| IBIS file generated by GenIBIS.pl Version 3.07
|   am35xxzer
[IBIS ver]   4.1
[File name]   sprm504.ibs
[File Rev]   1.0
[Date]   Mon May 10, 2010, 10:47:13
[Source]   Data created at Texas Instruments
[Notes]   1) IBIS spec conformance checker (IBISCK4) ran with 0 errors
   and 179 warnings.  Warnings can be waived.
[Disclaimer] Please be aware that in the absence of a written agreement,
   Texas Instruments (TI) assumes no liability for: 1) the
   accuracy of the IBIS models provided to your company, 2) the
   proper functioning of these IBIS models in your design or for
   any resulting applications, or, 3) infringement of patents,
   copyrights, or intellectual property rights resulting from
   your use of these IBIS models. TI provides IBIS models as a
   service to our customers and therefore reserves the right to
   limit distribution of the IBIS models.
[Copyright]   Property of Texas Instruments Incorporated. Unauthorised
   reproduction and/or distribution is strictly prohibited. This
   product is protected under copyright law and trade secret law
   as an unpublished work. Created 2010,(C) Copyright 2010,
   Texas Instruments Incorporated., All Rights Reserved. These
   commodities are under the U.S. Government distribution license
   control.As such,they are not to be re-exported without the
   prior approval of the U.S. Department of Commerce.
|   Component am35xxzer
[Component]   am35xxzer
[Manufacturer]   Texas Instruments.
[Package]
|   typ   min   max
R_pkg   0.33395   214.1400E-3   453.7600E-3
L_pkg   6.28345E-009   3.3793E-9   9.1876E-9
C_pkg   2.39255E-012   1.3394E-12   3.4457E-12
[Pin]   signal_name   model_name   R_pin   L_pin   C_pin
A2   MCBSP4_DX   Selector_25  394.1900E-3 7.9895E-9  1.9401E-12
A3   MCBSP4_CLKX   Selector_25  371.6000E-3 7.7376E-9  1.9311E-12
A4   MCBSP3_FSX   Selector_25  347.7300E-3 7.0891E-9  2.0982E-12
A5   UART2_CTS   Selector_12  328.5900E-3 6.4462E-9  1.5188E-12
A7   USB0_DRVVBUS   Selector_9   336.2200E-3 6.8852E-9  1.6105E-12
A8   SYS_32K   Selector_17  296.9800E-3 5.8091E-9  1.6649E-12
A10   SYS_XTALIN   Selector_11  282.6900E-3 5.0981E-9  1.6542E-12
A12   JTAG_TMS_TMSC   Selector_14  324.6800E-3 6.3416E-9  1.5318E-12
A13   DSS_DATA20   Selector_8   341.4400E-3 6.7413E-9  1.6482E-12
A14   DSS_DATA17   Selector_8   333.0200E-3 6.8421E-9  1.5875E-12
A15   DSS_DATA16   Selector_8   314.2700E-3 6.1729E-9  1.5039E-12
A16   DSS_DATA13   Selector_8   297.6500E-3 5.9252E-9  1.5015E-12
A17   DSS_DATA4   Selector_25  346.9100E-3 7.2431E-9  1.7900E-12
A18   DSS_DATA2   Selector_25  329.7600E-3 6.8073E-9  1.6863E-12
A19   DSS_DATA1   Selector_25  330.6900E-3 6.8826E-9  1.7355E-12
A20   DSS_DATA0   Selector_25  315.8500E-3 6.5578E-9  1.8340E-12
AA2   SDRC_D28   Selector_16  343.2000E-3 6.9062E-9  1.8222E-12
AA3   SDRC_D29   Selector_16  324.2800E-3 6.4573E-9  1.8291E-12
AA4   SDRC_D30   Selector_16  316.2700E-3 6.3226E-9  1.7135E-12
AA5   GPMC_A4   Selector_2   329.6700E-3 6.0019E-9  1.5140E-12
AA6   GPMC_A7   Selector_27  298.1300E-3 6.0001E-9  1.5038E-12
AA7   GPMC_D0   Selector_27  320.6800E-3 6.0389E-9  1.5462E-12
AA8   GPMC_D5   Selector_27  323.1800E-3 5.8436E-9  1.5422E-12
AA9   GPMC_D3   Selector_27  380.0900E-3 7.6125E-9  1.7128E-12
AA10   GPMC_D12   Selector_27  301.4100E-3 5.4391E-9  1.4352E-12
AA11   GPMC_NCS4   Selector_27  374.8300E-3 7.1356E-9  1.5639E-12
AA12   GPMC_NCS6   Selector_27  374.6200E-3 7.0731E-9  1.6544E-12
AA13   UART3_RX_IRRX   Selector_18  314.2500E-3 5.8029E-9  1.6148E-12
AA14   GPMC_NADV_ALE   Selector_20  353.2500E-3 6.2559E-9  1.6326E-12
AA15   GPMC_NWE   Selector_21  385.0100E-3 7.2004E-9  1.5876E-12
AA16   GPMC_WAIT1   Selector_22  399.6800E-3 7.9386E-9  1.7244E-12
AA17   I2C1_SCL   Selector_7   370.5100E-3 7.2651E-9  1.7713E-12
AA18   SYS_NRESPWRON   Selector_23  360.3900E-3 7.0919E-9  1.8556E-12
AA19   SYS_BOOT3   Selector_26  384.4600E-3 7.6592E-9  1.9352E-12
AA20   SYS_BOOT7   Selector_24  393.7300E-3 7.7930E-9  1.9516E-12
AA21   CCDC_FIELD   Selector_25  398.4600E-3 8.0595E-9  2.0452E-12
AB2   SDRC_D31   Selector_16  334.8800E-3 7.1146E-9  1.7302E-12
AB3   SDRC_DM3   Selector_28  329.7900E-3 6.8551E-9  1.7153E-12
AB4   GPMC_A3   Selector_2   347.2000E-3 6.7527E-9  1.4825E-12
AB5   GPMC_A5   Selector_2   343.8700E-3 6.4609E-9  1.5166E-12
AB6   GPMC_A6   Selector_27  346.1000E-3 6.4915E-9  1.5619E-12
AB7   GPMC_A9   Selector_27  311.5600E-3 6.3969E-9  1.5303E-12
AB8   GPMC_D6   Selector_27  330.3400E-3 6.2412E-9  1.3398E-12
AB9   GPMC_D9   Selector_27  338.5000E-3 6.5927E-9  1.4492E-12
AB10   GPMC_D10   Selector_27  337.0400E-3 6.2083E-9  1.5036E-12
AB13   GPMC_CLK   Selector_6   355.3300E-3 6.5540E-9  1.5066E-12
AB14   GPMC_NOE   Selector_21  335.0300E-3 6.5910E-9  1.4501E-12
AB15   HECC1_TXD   Selector_18  342.7600E-3 5.8516E-9  1.4047E-12
AB16   HECC1_RXD   Selector_18  364.8600E-3 7.0099E-9  1.4836E-12
AB17   I2C1_SDA   Selector_7   374.5600E-3 7.3256E-9  1.6503E-12
AB18   SYS_NIRQ   Selector_18  393.1800E-3 7.5773E-9  1.7479E-12
AB19   SYS_BOOT0   Selector_26  401.5700E-3 8.1494E-9  1.7968E-12
AB20   SYS_BOOT1   Selector_26  403.8500E-3 8.2825E-9  1.9344E-12
AB21   CCDC_PCLK   Selector_25  387.0200E-3 7.9369E-9  2.0262E-12
B2   MCBSP4_FSX   Selector_25  387.3500E-3 8.1272E-9  1.9226E-12
B3   MCBSP4_DR   Selector_25  356.5700E-3 6.6431E-9  3.4457E-12
B4   MCBSP3_DR   Selector_25  337.2600E-3 6.7319E-9  1.7321E-12
B5   UART2_RTS   Selector_12  315.8800E-3 6.1959E-9  1.5252E-12
B8   SYS_CLKREQ   Selector_5   411.2600E-3 8.1051E-9  1.9939E-12
B9   HDQ_SIO   Selector_14  357.0800E-3 6.9052E-9  1.7073E-12
B11   MCBSP1_CLKR   Selector_8   346.6900E-3 6.8467E-9  1.6577E-12
B12   JTAG_TDI   Selector_15  314.3500E-3 5.8609E-9  1.6005E-12
B13   DSS_DATA21   Selector_8   337.3800E-3 6.4124E-9  1.6594E-12
B14   DSS_DATA23   Selector_8   266.3400E-3 5.2657E-9  1.4591E-12
B15   DSS_DATA15   Selector_8   347.3200E-3 6.9786E-9  1.6179E-12
B16   DSS_DATA7   Selector_8   334.0200E-3 7.2239E-9  1.7318E-12
B17   DSS_DATA8   Selector_8   310.1100E-3 6.1300E-9  1.5935E-12
B18   DSS_DATA3   Selector_25  310.5900E-3 6.3123E-9  1.6778E-12
B19   DSS_ACBIAS   Selector_25  323.0400E-3 6.4094E-9  1.7859E-12
B20   DSS_VSYNC   Selector_12  331.2700E-3 6.6497E-9  1.8950E-12
B21   DSS_HSYNC   Selector_12  352.7100E-3 7.2376E-9  2.0639E-12
B22   DSS_PCLK   Selector_12  371.9600E-3 8.0470E-9  2.0412E-12
C1   SDRC_D6   Selector_16  387.7900E-3 7.7181E-9  2.0792E-12
C2   SDRC_D3   Selector_16  391.4300E-3 7.8287E-9  1.9588E-12
C3   SDRC_D2   Selector_16  364.3000E-3 7.1726E-9  2.2255E-12
C4   MCBSP3_DX   Selector_25  294.3600E-3 5.9515E-9  1.8296E-12
C5   MCBSP2_DR   Selector_25  298.3000E-3 5.8783E-9  2.2622E-12
C6   UART2_RX   Selector_12  250.8400E-3 4.7866E-9  1.5785E-12
C8   MCBSP1_CLKX   Selector_8   377.9200E-3 7.4558E-9  1.8963E-12
C9   MCBSP1_DR   Selector_8   389.9800E-3 8.0809E-9  1.9704E-12
C10   MCBSP1_DX   Selector_8   353.0200E-3 7.4383E-9  1.7696E-12
C11   MCBSP1_FSX   Selector_8   281.2900E-3 5.3536E-9  1.6619E-12
C12   JTAG_RTCK   Selector_1   322.1600E-3 6.1913E-9  1.7196E-12
C13   DSS_DATA18   Selector_8   341.7000E-3 7.0786E-9  1.8615E-12
C14   DSS_DATA22   Selector_8   294.8300E-3 5.3265E-9  1.6648E-12
C15   DSS_DATA19   Selector_8   323.1600E-3 6.1811E-9  1.6720E-12
C16   DSS_DATA10   Selector_8   236.1700E-3 4.0981E-9  1.5175E-12
C17   DSS_DATA9   Selector_8   281.6200E-3 5.4065E-9  1.5927E-12
C18   DSS_DATA5   Selector_25  278.8000E-3 5.7416E-9  1.7921E-12
C19   UART1_CTS   Selector_25  330.0200E-3 6.6620E-9  2.1791E-12
C20   UART1_RX   Selector_25  309.1300E-3 6.3006E-9  2.0807E-12
C21   UART1_RTS   Selector_25  352.2800E-3 7.3603E-9  2.0641E-12
C22   UART1_TX   Selector_25  352.7900E-3 7.5858E-9  2.0647E-12
D1   SDRC_D7   Selector_16  382.6500E-3 7.6199E-9  1.8172E-12
D2   SDRC_D5   Selector_16  381.8600E-3 7.5301E-9  2.0289E-12
D3   SDRC_D1   Selector_16  367.9300E-3 7.3780E-9  1.9522E-12
D4   MCBSP3_CLKX   Selector_25  308.1500E-3 5.9447E-9  1.8755E-12
D5   MCBSP2_CLKX   Selector_25  281.9900E-3 5.4739E-9  1.7314E-12
D6   UART2_TX   Selector_12  257.7400E-3 4.4275E-9  1.5079E-12
D11   MCBSP1_FSR   Selector_8   369.7200E-3 7.2459E-9  1.9001E-12
D12   JTAG_TDO   Selector_1   265.2300E-3 4.5313E-9  1.7160E-12
D13   JTAG_NTRST   Selector_13  286.1200E-3 5.1160E-9  1.6364E-12
D14   DSS_DATA12   Selector_8   346.7700E-3 6.6345E-9  1.9652E-12
D15   DSS_DATA14   Selector_8   258.7600E-3 4.2155E-9  1.9942E-12
D16   DSS_DATA11   Selector_8   241.9700E-3 4.1793E-9  1.4888E-12
D17   DSS_DATA6   Selector_8   266.8500E-3 4.8979E-9  1.8781E-12
D18   ETK_D15   Selector_25  377.1800E-3 7.5826E-9  2.1548E-12
D19   ETK_D14   Selector_25  441.6100E-3 9.1469E-9  2.3614E-12
D20   ETK_D13   Selector_25  378.0400E-3 7.6774E-9  2.1153E-12
D21   ETK_D9   Selector_8   386.7400E-3 8.1228E-9  1.9629E-12
D22   ETK_D8   Selector_8   332.1700E-3 7.1693E-9  1.8447E-12
E1   SDRC_DQS0N   Selector_16  380.3600E-3 7.1982E-9  1.7436E-12
E2   SDRC_DQS0P   Selector_16  383.5300E-3 7.3006E-9  1.8495E-12
E3   SDRC_D0   Selector_16  370.1100E-3 6.9891E-9  1.8851E-12
E4   MCBSP2_DX   Selector_25  262.2800E-3 4.7706E-9  1.8633E-12
E5   MCBSP2_FSX   Selector_25  260.4900E-3 4.6931E-9  1.7057E-12
E9   SYS_CLKOUT1   Selector_14  363.2700E-3 6.8582E-9  2.0365E-12
E10   SYS_CLKOUT2   Selector_5   297.2300E-3 4.8817E-9  1.9430E-12
E11   MCBSP_CLKS   Selector_8   269.9100E-3 4.5189E-9  1.8433E-12
E12   JTAG_EMU1   Selector_14  261.5900E-3 4.3757E-9  1.7218E-12
E13   JTAG_EMU0   Selector_14  214.1400E-3 3.3793E-9  1.6303E-12
E14   JTAG_TCK   Selector_13  245.4800E-3 3.8516E-9  1.8426E-12
E18   ETK_D12   Selector_25  376.9800E-3 7.5870E-9  2.0810E-12
E19   ETK_D4   Selector_8   417.7500E-3 9.0359E-9  2.2165E-12
E20   ETK_D11   Selector_8   286.1400E-3 6.0147E-9  1.7651E-12
E21   ETK_D7   Selector_8   332.2800E-3 6.5712E-9  1.8104E-12
E22   ETK_D10   Selector_8   332.0100E-3 6.6808E-9  1.6882E-12
F1   SDRC_STRBEN_DLY0   Selector_16  345.4800E-3 7.0094E-9  1.6124E-12
F2   SDRC_STRBEN0   Selector_3   397.3300E-3 7.7827E-9  1.7655E-12
F3   SDRC_D4   Selector_16  377.3600E-3 7.2235E-9  1.9370E-12
F4   SDRC_DM0   Selector_28  376.8400E-3 6.7876E-9  1.9715E-12
F19   ETK_D6   Selector_8   358.0800E-3 7.6020E-9  2.0805E-12
F20   ETK_D2   Selector_4   390.0700E-3 8.3332E-9  1.9946E-12
F21   ETK_D5   Selector_8   318.2400E-3 6.4677E-9  1.6886E-12
F22   ETK_D1   Selector_4   335.7100E-3 7.2115E-9  1.7000E-12
G1   SDRC_D13   Selector_16  371.0000E-3 7.3116E-9  1.5578E-12
G2   SDRC_D8   Selector_16  347.1200E-3 6.6314E-9  1.5883E-12
G3   SDRC_D9   Selector_16  365.8200E-3 6.7223E-9  1.6945E-12
G4   SDRC_D11   Selector_16  357.6800E-3 6.3782E-9  1.6674E-12
G19   ETK_D3   Selector_8   358.3200E-3 7.2960E-9  1.9773E-12
G20   ETK_D0   Selector_4   333.3800E-3 6.3463E-9  1.8362E-12
G21   ETK_CTL   Selector_4   355.8700E-3 7.1967E-9  1.7778E-12
G22   ETK_CLK   Selector_4   325.5100E-3 6.5023E-9  1.5883E-12
H1   SDRC_DQS1N   Selector_16  350.2100E-3 6.1171E-9  1.5409E-12
H2   SDRC_DQS1P   Selector_16  347.4900E-3 6.2728E-9  1.5909E-12
H3   SDRC_D10   Selector_16  360.1200E-3 6.6289E-9  1.6396E-12
H4   SDRC_D12   Selector_16  354.7800E-3 6.2968E-9  2.0266E-12
H19   MCSPI2_CS1   Selector_8   393.8600E-3 8.0415E-9  1.9650E-12
H20   MCSPI2_SIMO   Selector_8   368.8400E-3 7.3875E-9  1.7931E-12
H21   MCSPI2_CS0   Selector_4   279.6000E-3 5.2827E-9  1.6108E-12
H22   MCSPI2_SOMI   Selector_8   319.4400E-3 6.4433E-9  1.5465E-12
J1   SDRC_D15   Selector_16  348.4000E-3 6.7968E-9  1.4180E-12
J2   SDRC_DM1   Selector_28  371.3300E-3 7.2561E-9  1.5449E-12
J3   SDRC_D14   Selector_16  331.4100E-3 6.0209E-9  1.6142E-12
J4   SDRC_NCS0   Selector_28  352.5300E-3 6.6031E-9  2.0882E-12
J5   SDRC_BA2   Selector_28  347.8200E-3 6.1291E-9  1.8458E-12
J18   MCSPI1_SOMI   Selector_25  437.3800E-3 9.1876E-9  2.1726E-12
J19   MCSPI1_CS2   Selector_4   309.3500E-3 5.8088E-9  1.7548E-12
J20   MCSPI1_CS1   Selector_12  371.9300E-3 7.8538E-9  1.8360E-12
J21   MCSPI1_CS3   Selector_4   298.0900E-3 5.8232E-9  1.5067E-12
J22   MCSPI2_CLK   Selector_8   292.2000E-3 6.0361E-9  1.4963E-12
K1   SDRC_NRAS   Selector_28  342.3100E-3 6.2301E-9  1.3738E-12
K2   SDRC_NWE   Selector_28  345.7800E-3 6.2263E-9  1.4739E-12
K3   SDRC_CKE0   Selector_28  349.0500E-3 6.3435E-9  1.5767E-12
K4   SDRC_NCS1   Selector_28  315.1600E-3 5.1791E-9  1.7620E-12
K5   SDRC_BA1   Selector_28  346.3100E-3 6.4474E-9  1.8052E-12
K18   MCSPI1_CS0   Selector_12  403.2100E-3 7.6981E-9  2.1120E-12
K19   MCSPI1_SIMO   Selector_25  295.7200E-3 5.6746E-9  1.7458E-12
K20   MMC2_DAT0   Selector_12  384.8200E-3 8.0396E-9  1.9443E-12
K21   MMC2_DAT3   Selector_12  364.1900E-3 7.3812E-9  1.7320E-12
K22   MCSPI1_CLK   Selector_25  319.3600E-3 6.4116E-9  1.5303E-12
L1   SDRC_CLK   Selector_28  331.5100E-3 5.8650E-9  1.3596E-12
L2   SDRC_NCLK   Selector_28  324.5300E-3 5.3251E-9  1.4459E-12
L3   SDRC_NCAS   Selector_28  298.6500E-3 4.6001E-9  1.4120E-12
L4   SDRC_BA0   Selector_28  327.7000E-3 5.5509E-9  1.9863E-12
L18   MMC2_DAT4   Selector_25  302.4100E-3 5.4584E-9  1.7910E-12
L19   MMC2_DAT1   Selector_12  322.0900E-3 5.8832E-9  1.7879E-12
L20   MMC2_DAT5   Selector_25  285.9200E-3 5.4253E-9  1.6563E-12
L21   MMC2_DAT6   Selector_25  299.2000E-3 5.9395E-9  1.5026E-12
M3   SDRC_A0   Selector_28  298.7800E-3 4.7878E-9  1.3523E-12
M4   SDRC_A1   Selector_28  299.2400E-3 4.5715E-9  1.7576E-12
M5   SDRC_A2   Selector_28  309.8900E-3 4.9618E-9  1.5021E-12
M18   MMC2_DAT2   Selector_12  268.7900E-3 4.2257E-9  1.7734E-12
M19   MMC2_DAT7   Selector_25  251.1900E-3 4.2376E-9  1.5452E-12
M20   MMC2_CMD   Selector_12  332.9000E-3 6.3877E-9  1.7093E-12
M21   MMC2_CLK   Selector_25  345.8900E-3 7.0265E-9  1.6777E-12
N2   SDRC_A4   Selector_28  319.1200E-3 5.9130E-9  1.3973E-12
N3   SDRC_A3   Selector_28  298.2300E-3 5.0225E-9  1.4214E-12
N4   SDRC_A5   Selector_28  292.3500E-3 4.7242E-9  1.4608E-12
N18   MMC1_DAT6   Selector_25  281.3200E-3 4.9560E-9  1.7518E-12
N19   MMC1_DAT5   Selector_25  300.7200E-3 5.4292E-9  1.6801E-12
N20   MMC1_DAT1   Selector_25  368.1700E-3 7.3968E-9  1.8328E-12
N21   MMC1_CMD   Selector_25  369.8200E-3 7.5325E-9  1.7934E-12
N22   MMC1_DAT4   Selector_25  316.1800E-3 6.3428E-9  1.5237E-12
P1   SDRC_A8   Selector_28  333.9700E-3 6.3888E-9  1.3394E-12
P2   SDRC_A7   Selector_28  300.4800E-3 5.2436E-9  1.3626E-12
P3   SDRC_A6   Selector_28  391.3500E-3 7.6328E-9  1.6789E-12
P4   SDRC_A9   Selector_28  288.7200E-3 4.5390E-9  1.4523E-12
P18   MMC1_DAT7   Selector_25  239.3400E-3 3.7935E-9  1.5614E-12
P19   MMC1_DAT2   Selector_25  319.3500E-3 6.0435E-9  1.8933E-12
P20   MMC1_DAT3   Selector_25  274.2200E-3 5.1565E-9  1.6198E-12
P21   MMC1_DAT0   Selector_25  287.1000E-3 5.8785E-9  1.6440E-12
P22   MMC1_CLK   Selector_25  332.4500E-3 6.4927E-9  1.6354E-12
R1   SDRC_A10   Selector_28  332.9700E-3 6.2895E-9  1.3521E-12
R2   SDRC_A11   Selector_28  302.8600E-3 5.4700E-9  1.4205E-12
R3   SDRC_A12   Selector_28  335.0100E-3 6.1858E-9  1.6138E-12
R4   SDRC_A13   Selector_28  286.1300E-3 4.4509E-9  1.4903E-12
R19   RMII_TXEN   Selector_12  258.9000E-3 4.3779E-9  1.7140E-12
R20   RMII_TXD1   Selector_12  345.4200E-3 6.6547E-9  1.8280E-12
R21   RMII_50MHZ_CLK   Selector_12  310.9600E-3 5.9238E-9  1.6144E-12
R22   RMII_RXER   Selector_12  297.6700E-3 6.0140E-9  1.6094E-12
T1   SDRC_ODT0   Selector_3   340.4300E-3 6.5941E-9  1.4560E-12
T2   SDRC_A14   Selector_28  373.1900E-3 7.0944E-9  1.6927E-12
T3   SDRC_D16   Selector_16  358.7500E-3 6.4974E-9  1.6588E-12
T4   SDRC_DM2   Selector_28  372.2700E-3 7.0453E-9  1.7643E-12
T19   RMII_RXD0   Selector_12  407.7500E-3 8.6597E-9  2.1127E-12
T20   RMII_RXD1   Selector_12  374.4500E-3 7.5508E-9  1.7800E-12
T21   RMII_CRS_DV   Selector_12  348.4500E-3 6.9689E-9  1.6427E-12
T22   RMII_TXD0   Selector_12  319.9300E-3 6.3790E-9  1.4976E-12
U1   SDRC_DQS2P   Selector_16  371.7300E-3 6.9258E-9  1.7011E-12
U2   SDRC_DQS2N   Selector_16  370.4900E-3 6.9212E-9  1.7419E-12
U3   SDRC_D17   Selector_16  391.3000E-3 7.7804E-9  1.7034E-12
U4   SDRC_D18   Selector_16  362.2700E-3 6.5640E-9  1.7278E-12
U19   CCDC_DATA7   Selector_25  277.4700E-3 4.7688E-9  1.7684E-12
U20   CCDC_DATA5   Selector_25  321.0700E-3 6.1811E-9  2.0111E-12
U21   RMII_MDIO_DATA   Selector_12  322.8800E-3 6.5133E-9  1.8319E-12
U22   RMII_MDIO_CLK   Selector_12  334.1000E-3 6.4537E-9  1.6931E-12
V1   SDRC_D20   Selector_16  350.0000E-3 6.4475E-9  1.6431E-12
V2   SDRC_D21   Selector_16  348.3500E-3 6.3864E-9  1.6964E-12
V3   SDRC_D23   Selector_16  354.7800E-3 6.4040E-9  1.7637E-12
V4   SDRC_D19   Selector_16  350.2600E-3 6.4026E-9  1.8971E-12
V5   SDRC_D22   Selector_16  364.8700E-3 6.1162E-9  2.1147E-12
V9   GPMC_D15   Selector_27  288.9600E-3 4.4115E-9  2.0013E-12
V10   GPMC_D14   Selector_27  298.6500E-3 4.6276E-9  1.8153E-12
V11   GPMC_NCS7   Selector_27  260.0800E-3 3.5996E-9  1.6939E-12
V12   GPMC_NCS3   Selector_27  300.6900E-3 5.0402E-9  2.5815E-12
V13   GPMC_WAIT0   Selector_19  318.5900E-3 5.2779E-9  1.7424E-12
V14   GPMC_WAIT3   Selector_22  323.4400E-3 5.5129E-9  2.2233E-12
V18   SYS_BOOT4   Selector_26  381.9200E-3 6.3636E-9  2.3826E-12
V19   CCDC_DATA3   Selector_25  346.6300E-3 6.9222E-9  2.1706E-12
V20   CCDC_DATA6   Selector_25  293.5100E-3 5.4832E-9  1.8028E-12
V21   CCDC_DATA2   Selector_25  348.0800E-3 6.8155E-9  1.9451E-12
V22   CCDC_DATA4   Selector_25  358.9600E-3 7.3363E-9  1.9845E-12
W1   SDRC_STRBEN1   Selector_3   358.9000E-3 7.3389E-9  1.6439E-12
W2   SDRC_STRBEN_DLY1   Selector_16  335.3200E-3 6.5553E-9  1.6701E-12
W3   SDRC_D24   Selector_16  325.5700E-3 6.1775E-9  1.8469E-12
W4   SDRC_D25   Selector_16  314.6500E-3 5.9870E-9  1.8646E-12
W5   GPMC_A1   Selector_2   276.8000E-3 5.0254E-9  1.5121E-12
W6   GPMC_A8   Selector_27  285.8700E-3 4.8998E-9  1.5288E-12
W7   GPMC_D2   Selector_27  276.4000E-3 4.6134E-9  1.4322E-12
W8   GPMC_D7   Selector_27  277.9400E-3 4.6812E-9  1.3884E-12
W9   GPMC_D11   Selector_27  320.6500E-3 5.3436E-9  1.5758E-12
W10   GPMC_D8   Selector_27  374.2600E-3 6.9728E-9  1.8939E-12
W11   GPMC_NBE0_CLE   Selector_2   321.4900E-3 5.0429E-9  1.8791E-12
W12   GPMC_NCS5   Selector_27  346.3800E-3 6.0427E-9  1.6861E-12
W13   UART3_RTS_SD   Selector_18  397.9700E-3 7.4481E-9  1.9605E-12
W14   GPMC_NWP   Selector_2   348.5900E-3 5.4377E-9  2.0172E-12
W15   UART3_CTS_RCTX   Selector_14  453.7600E-3 9.0375E-9  2.0383E-12
W16   I2C3_SCL   Selector_10  426.9500E-3 8.4105E-9  2.0565E-12
W17   I2C3_SDA   Selector_10  425.3500E-3 8.1716E-9  2.0454E-12
W18   SYS_BOOT2   Selector_26  349.5100E-3 6.8866E-9  2.2001E-12
W19   SYS_BOOT6   Selector_26  354.7200E-3 7.1891E-9  2.2438E-12
W20   CCDC_DATA1   Selector_25  372.5000E-3 7.5019E-9  2.0839E-12
W21   CCDC_WEN   Selector_25  380.8600E-3 7.5639E-9  2.0544E-12
W22   CCDC_DATA0   Selector_25  364.7100E-3 7.6283E-9  2.1897E-12
Y1   SDRC_DQS3P   Selector_16  338.1200E-3 6.7375E-9  1.7844E-12
Y2   SDRC_DQS3N   Selector_16  334.6400E-3 6.5923E-9  1.8172E-12
Y3   SDRC_D26   Selector_16  320.0400E-3 6.0288E-9  1.8113E-12
Y4   SDRC_D27   Selector_16  308.9600E-3 5.8063E-9  1.9148E-12
Y5   GPMC_A2   Selector_2   304.6500E-3 5.6279E-9  1.5637E-12
Y6   GPMC_A10   Selector_27  300.8500E-3 5.4940E-9  1.4479E-12
Y7   GPMC_D1   Selector_27  300.0700E-3 5.4664E-9  1.4940E-12
Y8   GPMC_D4   Selector_27  279.2400E-3 5.0923E-9  1.6258E-12
Y9   GPMC_D13   Selector_27  279.2600E-3 4.4325E-9  1.3653E-12
Y10   GPMC_NCS0   Selector_27  300.7900E-3 5.1738E-9  1.3890E-12
Y11   GPMC_NCS1   Selector_27  393.9900E-3 7.7589E-9  1.7258E-12
Y12   GPMC_NCS2   Selector_27  409.1800E-3 8.0012E-9  1.7587E-12
Y13   UART3_TX_IRTX   Selector_18  334.1300E-3 5.7358E-9  1.4750E-12
Y14   GPMC_WAIT2   Selector_22  316.2000E-3 5.4373E-9  1.6324E-12
Y15   GPMC_NBE1   Selector_2   376.7200E-3 6.5308E-9  1.6988E-12
Y16   I2C2_SDA   Selector_10  379.4400E-3 6.9005E-9  1.9052E-12
Y17   I2C2_SCL   Selector_10  431.0600E-3 8.4745E-9  1.9947E-12
Y18   SYS_NRESWARM   Selector_9   413.4500E-3 7.9651E-9  2.0143E-12
Y19   SYS_BOOT5   Selector_26  364.3900E-3 6.8897E-9  1.9288E-12
Y20   SYS_BOOT8   Selector_24  378.6800E-3 7.4205E-9  2.0300E-12
Y21   CCDC_HD   Selector_25  376.1800E-3 7.3947E-9  1.9975E-12
Y22   CCDC_VD   Selector_25  388.2000E-3 7.9599E-9  2.0544E-12
| Device pads which are not required to be modeled. Included for completeness
|A1   VSS   VSS.PAD
|A6   USB0_DP   COMPLEXIO.PAD
|A9   SYS_XTALOUT   OOSCHF18CVS_7LM.PAD
|A11   VSS   VSS.PAD
|A21   VDDSHV   VDD.PAD
|A22   VSS   VSS.PAD
|AA1   VDDS   VDD.PAD
|AA22   VDDSHV   VDD.PAD
|AB1   VSS   VSS.PAD
|AB11   VDDSHV   VDD.PAD
|AB12   VSS   VSS.PAD
|AB22   VSS   VSS.PAD
|B1   VDDSHV   VDD.PAD
|B6   USB0_DM   COMPLEXIO.PAD
|B7   USB0_ID   COMPLEXIO.PAD
|B10   VSSOSC   VSS.PAD
|C7   USB0_VBUS   COMPLEXIO.PAD
|D7   VDDA1P8V_USBPHY   VDD.PAD
|E6   VSS   VSS.PAD
|E7   CAP_VDDA1P2LDO_USBPHY PASSIVE.PAD
|E15   VDDSHV   VDD.PAD
|E16   VSS   VSS.PAD
|E17   VDDSHV   VDD.PAD
|F5   VDDS   VDD.PAD
|F6   VSS   VSS.PAD
|F7   VDDA3P3V_USBPHY   VDD.PAD
|F11   VDDS_DPLL_PER_CORE   VDD.PAD
|F12   VDDSHV   VDD.PAD
|F13   VSS   VSS.PAD
|F14   VDDSHV   VDD.PAD
|F15   VSS   VSS.PAD
|F16   VDDS   VDD.PAD
|F17   VSS   VSS.PAD
|F18   VDDSHV   VDD.PAD
|G5   VSS   VSS.PAD
|G7   VSS   VSS.PAD
|G8   VDDSHV   VDD.PAD
|G9   VDDSOSC   VDD.PAD
|G10   VDDSHV   VDD.PAD
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[Model Selector] Selector_1
Model_10 I/O,3.3V,PD
Model_11 I/O,3.3V,PU
Model_12 I/O,3.3V,PI
Model_7 I/O,1.8V,PD
Model_8 I/O,1.8V,PU
Model_9 I/O,1.8V,PI
|   Usage IO#1.8V/3.3V#PD/PI/PU##BQ1833DV40DTPBFZP18LL_7LM_X50.PAD
|   Base model BQ1833DV40DTPBFZP18LL_7LM_X50
[Model Selector] Selector_2
Model_56 I/O,1.8V,PD
Model_57 I/O,1.8V,PU
Model_58 I/O,1.8V,PI
Model_59 I/O,3.3V,PD
Model_60 I/O,3.3V,PU
Model_61 I/O,3.3V,PI
|   Usage IO#1.8V#NONE_LVCMOS#FAST#BSSTL18TCSCGPBFZ_7LM.PAD
|   Base model BSSTL18TCSCGPBFZ_7LM
[Model Selector] Selector_3
Model_102 3-STATE,1.8V,PI,FAST,+-10%V
Model_105 INPUT,1.8V,NONE_LVCMOS,+-10%V
Model_115 3-STATE,1.8V,PI,FAST,+-0.1V
Model_118 INPUT,1.8V,NONE_LVCMOS,+-0.1V
|   Usage IO#1.8V/3.3V#PD/PI/PU##BC1833DV40CTPBFHP18LL_7LM.PAD
|   Base model BC1833DV40CTPBFHP18LL_7LM
[Model Selector] Selector_4
Model_1 I/O,1.8V,PD
Model_2 I/O,1.8V,PU
Model_3 I/O,1.8V,PI
Model_4 I/O,3.3V,PD
Model_5 I/O,3.3V,PU
Model_6 I/O,3.3V,PI
|   Usage IO#1.8V/3.3V#PD/PI/PU##BC1833DV50BTPBFZP18LL_7LM.PAD
|   Base model BC1833DV50BTPBFZP18LL_7LM
[Model Selector] Selector_5
Model_10 I/O,3.3V,PD
Model_11 I/O,3.3V,PU
Model_12 I/O,3.3V,PI
Model_7 I/O,1.8V,PD
Model_8 I/O,1.8V,PU
Model_9 I/O,1.8V,PI
|   Usage IO#1.8V/3.3V#PD/PI/PU##BQ1833DV40DTPBFZP18LL_7LM.PAD
|   Base model BQ1833DV40DTPBFZP18LL_7LM
[Model Selector] Selector_6
Model_31 I/O,1.8V,PD
Model_32 I/O,1.8V,PU
Model_33 I/O,1.8V,PI
Model_34 I/O,3.3V,PD
Model_35 I/O,3.3V,PU
Model_36 I/O,3.3V,PI
|   Usage OD#1.8V/3.3V#PD/PI/PU##BC1833DV65ATPBFHP18LL_7LM_X50.PAD
|   Base model BC1833DV65ATPBFHP18LL_7LM_X50
[Model Selector] Selector_7
Model_19 I/O,1.8V,PD
Model_20 I/O,1.8V,PU
Model_21 I/O,1.8V,PI
Model_22 I/O,3.3V,PD
Model_23 I/O,3.3V,PU
Model_24 I/O,3.3V,PI
|   Usage IO#1.8V/3.3V#PD/PI/PU##BC1833DV40CTPBFZP18LL_7LM.PAD
|   Base model BC1833DV40CTPBFZP18LL_7LM
[Model Selector] Selector_8
Model_76 I/O,1.8V,PD
Model_77 I/O,1.8V,PU
Model_78 I/O,1.8V,PI
Model_79 I/O,3.3V,PD
Model_80 I/O,3.3V,PU
Model_81 I/O,3.3V,PI
|   Usage IO#1.8V/3.3V#PD/PI/PU##BC1833DV50BTPBFZP18LL_7LM_X50.PAD
|   Base model BC1833DV50BTPBFZP18LL_7LM_X50
[Model Selector] Selector_9
Model_94 I/O,1.8V,PD
Model_95 I/O,1.8V,PU
Model_96 I/O,1.8V,PI
Model_97 I/O,3.3V,PD
Model_98 I/O,3.3V,PU
Model_99 I/O,3.3V,PI
|   Usage IO#1.8V/3.3V#PD/PI/PU##BC1833DV65ATPBFHP18LL_7LM_X50.PAD
|   Base model BC1833DV65ATPBFHP18LL_7LM_X50
[Model Selector] Selector_10
Model_19 I/O,1.8V,PD
Model_20 I/O,1.8V,PU
Model_21 I/O,1.8V,PI
Model_22 I/O,3.3V,PD
Model_23 I/O,3.3V,PU
Model_24 I/O,3.3V,PI
|   Usage I#1.8V###IOSCHF18CVSHY_7LM.PAD
|   Base model IOSCHF18CVSHY_7LM
[Model Selector] Selector_11
Model_37 INPUT,1.8V
|   Usage IO#1.8V/3.3V#PD/PI/PU##BC1833DV40CTPBFHP18LL_7LM_X50.PAD
|   Base model BC1833DV40CTPBFHP18LL_7LM_X50
[Model Selector] Selector_12
Model_70 I/O,1.8V,PD
Model_71 I/O,1.8V,PU
Model_72 I/O,1.8V,PI
Model_73 I/O,3.3V,PD
Model_74 I/O,3.3V,PU
Model_75 I/O,3.3V,PI
|   Usage I#1.8V/3.3V#PD/PI/PU##IC1833DVTPBFZP18LL_7LM.PAD
|   Base model IC1833DVTPBFZP18LL_7LM
[Model Selector] Selector_13
Model_13 INPUT,1.8V,PD
Model_14 INPUT,1.8V,PU
Model_15 INPUT,1.8V,PI
Model_16 INPUT,3.3V,PD
Model_17 INPUT,3.3V,PU
Model_18 INPUT,3.3V,PI
|   Usage IO#1.8V/3.3V#PD/PI/PU##BC1833DV50BTPBFHP18LL_7LM.PAD
|   Base model BC1833DV50BTPBFHP18LL_7LM
[Model Selector] Selector_14
Model_134 I/O,1.8V,PD
Model_135 I/O,1.8V,PU
Model_136 I/O,1.8V,PI
Model_137 I/O,3.3V,PD
Model_138 I/O,3.3V,PU
Model_139 I/O,3.3V,PI
|   Usage I#1.8V/3.3V#PD/PI/PU##IC1833DVTPBFHP18LL_7LM.PAD
|   Base model IC1833DVTPBFHP18LL_7LM
[Model Selector] Selector_15
Model_44 INPUT,1.8V,PD
Model_45 INPUT,1.8V,PU
Model_46 INPUT,1.8V,PI
Model_47 INPUT,3.3V,PD
Model_48 INPUT,3.3V,PU
Model_49 INPUT,3.3V,PI
|   Usage IO#1.8V#FULL_SSTL/HALF_SSTL/NONE_SSTL#FAST#BSSTL18TCSCGPBFZ_7LM.PAD
|   Base model BSSTL18TCSCGPBFZ_7LM
[Model Selector] Selector_16
Model_100 INPUT,1.8V,HALF_SSTL,+-10%V
Model_102 3-STATE,1.8V,PI,FAST,+-10%V
Model_104 INPUT,1.8V,FULL_SSTL,+-10%V
Model_107 INPUT,1.8V,NONE_SSTL,+-10%V
Model_113 INPUT,1.8V,HALF_SSTL,+-0.1V
Model_115 3-STATE,1.8V,PI,FAST,+-0.1V
Model_117 INPUT,1.8V,FULL_SSTL,+-0.1V
Model_120 INPUT,1.8V,NONE_SSTL,+-0.1V
|   Usage I#1.8V/3.3V#PD/PI/PU##IQ1833DVTPBFZP18LL_7LM.PAD
|   Base model IQ1833DVTPBFZP18LL_7LM
[Model Selector] Selector_17
Model_82 INPUT,1.8V,PD
Model_83 INPUT,1.8V,PU
Model_84 INPUT,1.8V,PI
Model_85 INPUT,3.3V,PD
Model_86 INPUT,3.3V,PU
Model_87 INPUT,3.3V,PI
|   Usage IO#1.8V/3.3V#PD/PI/PU##BC1833DV50BTPBFHP18LL_7LM_X50.PAD
|   Base model BC1833DV50BTPBFHP18LL_7LM_X50
[Model Selector] Selector_18
Model_62 I/O,1.8V,PD
Model_63 I/O,1.8V,PU
Model_64 I/O,1.8V,PI
Model_65 I/O,3.3V,PD
Model_66 I/O,3.3V,PU
Model_67 I/O,3.3V,PI
|   Usage I#1.8V/3.3V#PD/PI/PU##BQ1833DV40DTPBFHP18LL_7LM_X50.PAD
|   Base model BQ1833DV40DTPBFHP18LL_7LM_X50
[Model Selector] Selector_19
Model_50 I/O,1.8V,PD
Model_51 I/O,1.8V,PU
Model_52 I/O,1.8V,PI
Model_53 I/O,3.3V,PD
Model_54 I/O,3.3V,PU
Model_55 I/O,3.3V,PI
|   Usage O#1.8V/3.3V###BQ1833DV40DTPBFZP18LL_7LM_X50.PAD
|   Base model BQ1833DV40DTPBFZP18LL_7LM_X50
[Model Selector] Selector_20
Model_56 I/O,1.8V,PD
Model_57 I/O,1.8V,PU
Model_58 I/O,1.8V,PI
Model_59 I/O,3.3V,PD
Model_60 I/O,3.3V,PU
Model_61 I/O,3.3V,PI
|   Usage O#1.8V/3.3V###BQ1833DV40DTPBFHP18LL_7LM_X50.PAD
|   Base model BQ1833DV40DTPBFHP18LL_7LM_X50
[Model Selector] Selector_21
Model_50 I/O,1.8V,PD
Model_51 I/O,1.8V,PU
Model_52 I/O,1.8V,PI
Model_53 I/O,3.3V,PD
Model_54 I/O,3.3V,PU
Model_55 I/O,3.3V,PI
|   Usage IO#1.8V/3.3V#PD/PI/PU##BQ1833DV40DTPBFHP18LL_7LM_X50.PAD
|   Base model BQ1833DV40DTPBFHP18LL_7LM_X50
[Model Selector] Selector_22
Model_50 I/O,1.8V,PD
Model_51 I/O,1.8V,PU
Model_52 I/O,1.8V,PI
Model_53 I/O,3.3V,PD
Model_54 I/O,3.3V,PU
Model_55 I/O,3.3V,PI
|   Usage I#1.8V/3.3V###IHHV1833DVTP18_7LM.PAD
|   Base model IHHV1833DVTP18_7LM
[Model Selector] Selector_23
Model_68 INPUT,1.8V
Model_69 INPUT,3.3V
|   Usage I#1.8V/3.3V#PD/PI/PU##BQ1833DV50BTPBFZP18LL_7LM_X50.PAD
|   Base model BQ1833DV50BTPBFZP18LL_7LM_X50
[Model Selector] Selector_24
Model_88 I/O,1.8V,PD
Model_89 I/O,1.8V,PU
Model_90 I/O,1.8V,PI
Model_91 I/O,3.3V,PD
Model_92 I/O,3.3V,PU
Model_93 I/O,3.3V,PI
|   Usage IO#1.8V/3.3V#PD/PI/PU##BC1833DV40CTPBFZP18LL_7LM_X50.PAD
|   Base model BC1833DV40CTPBFZP18LL_7LM_X50
[Model Selector] Selector_25
Model_38 I/O,1.8V,PD
Model_39 I/O,1.8V,PU
Model_40 I/O,1.8V,PI
Model_41 I/O,3.3V,PD
Model_42 I/O,3.3V,PU
Model_43 I/O,3.3V,PI
|   Usage IO#1.8V/3.3V#PD/PI/PU##BQ1833DV50BTPBFZP18LL_7LM_X50.PAD
|   Base model BQ1833DV50BTPBFZP18LL_7LM_X50
[Model Selector] Selector_26
Model_88 I/O,1.8V,PD
Model_89 I/O,1.8V,PU
Model_90 I/O,1.8V,PI
Model_91 I/O,3.3V,PD
Model_92 I/O,3.3V,PU
Model_93 I/O,3.3V,PI
|   Usage IO#1.8V/3.3V#PD/PI/PU##BQ1833DV40DTPBFHP18LL_7LM.PAD
|   Base model BQ1833DV40DTPBFHP18LL_7LM
[Model Selector] Selector_27
Model_25 I/O,1.8V,PD
Model_26 I/O,1.8V,PU
Model_27 I/O,1.8V,PI
Model_28 I/O,3.3V,PD
Model_29 I/O,3.3V,PU
Model_30 I/O,3.3V,PI
|   Usage O#1.8V##FAST#BSSTL18TCSCGPBFZ_7LM.PAD
|   Base model BSSTL18TCSCGPBFZ_7LM
[Model Selector] Selector_28
Model_102 3-STATE,1.8V,PI,FAST,+-10%V
Model_115 3-STATE,1.8V,PI,FAST,+-0.1V
| Models and submodels in the file (115): Model_1 (I/O), Model_2 (I/O), Model_3 (I/O), Model_4 (I/O), Model_5 (I/O), Model_6 (I/O), Model_7 (I/O), Model_8 (I/O), Model_9 (I/O), Model_10 (I/O), Model_11 (I/O), Model_12 (I/O), Model_13 (Input), Model_14 (Input), Model_15 (Input), Model_16 (Input), Model_17 (Input), Model_18 (Input), Model_19 (I/O), Model_20 (I/O), Model_21 (I/O), Model_22 (I/O), Model_23 (I/O), Model_24 (I/O), Model_25 (I/O), Model_26 (I/O), Model_27 (I/O), Model_28 (I/O), Model_29 (I/O), Model_30 (I/O), Model_31 (I/O), Model_32 (I/O), Model_33 (I/O), Model_34 (I/O), Model_35 (I/O), Model_36 (I/O), Model_37 (Input), Model_38 (I/O), Model_39 (I/O), Model_40 (I/O), Model_41 (I/O), Model_42 (I/O), Model_43 (I/O), Model_44 (Input), Model_45 (Input), Model_46 (Input), Model_47 (Input), Model_48 (Input), Model_49 (Input), Model_50 (I/O), Model_51 (I/O), Model_52 (I/O), Model_53 (I/O), Model_54 (I/O), Model_55 (I/O), Model_56 (I/O), Model_57 (I/O), Model_58 (I/O), Model_59 (I/O), Model_60 (I/O), Model_61 (I/O), Model_62 (I/O), Model_63 (I/O), Model_64 (I/O), Model_65 (I/O), Model_66 (I/O), Model_67 (I/O), Model_68 (Input), Model_69 (Input), Model_70 (I/O), Model_71 (I/O), Model_72 (I/O), Model_73 (I/O), Model_74 (I/O), Model_75 (I/O), Model_76 (I/O), Model_77 (I/O), Model_78 (I/O), Model_79 (I/O), Model_80 (I/O)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
